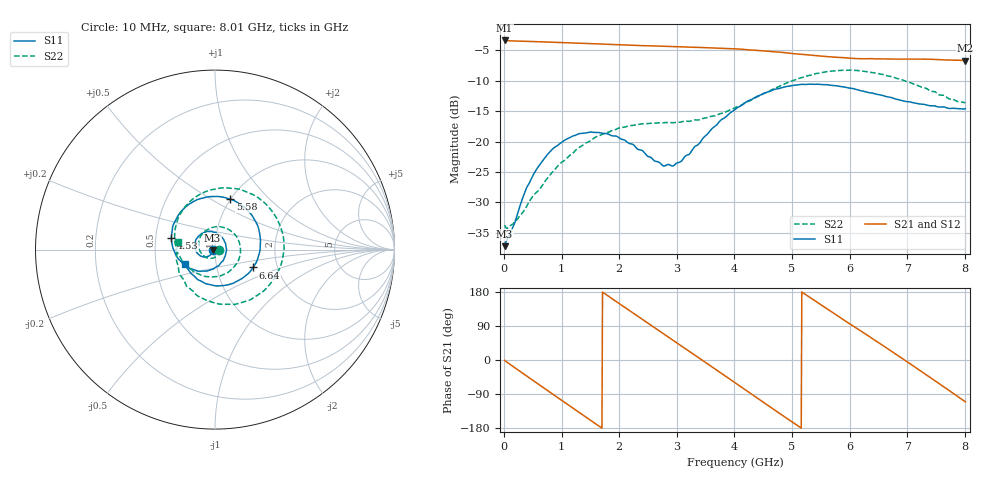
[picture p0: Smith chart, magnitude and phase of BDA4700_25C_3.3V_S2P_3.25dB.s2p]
!Agilent Technologies,E5071B,MY42404982,A.09.10
!Date: Mon Oct 20 18:04:20 2025
!Data & Calibration Information:
!Freq	S11:SOLT2(ON)	S21:SOLT2(ON)	S12:SOLT2(ON)	S22:SOLT2(ON)
# Hz S RI R 50
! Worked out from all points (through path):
!   801 points, 10 MHz to 8.01 GHz, reference 50 ohm
!   highest |S21| = -3.37 dB at 10 MHz (marker M1); lowest = -6.7 dB at 8.01 GHz (marker M2)
!   group delay of S21, straight-line fit = 287 ps
!   lowest |S11| = -37.2 dB at 10 MHz (marker M3), VSWR 1.03, Z = 48.6 - j0.153 ohm
!   |S11| at or under -10 dB: start of sweep to end of sweep
!   |S22| runs from -34.3 to -8.2 dB; largest |S21 - S12| = 0.0077
!   S11 on the Smith chart (normalised r, x): 10 MHz: 0.97, -0.00; 4.53 GHz: 0.60, +0.08; 5.58 GHz: 1.00, +0.61; 6.64 GHz: 1.50, -0.32; 8.01 GHz: 0.70, -0.12
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1e7  -0.0137 -0.00158  0.6786 -0.0146  0.6784 -0.0151  0.0205 -0.0018
3.3e8  -0.0228 -0.0266  0.5442 -0.3886  0.5438 -0.3889  0.019 -0.0182
7.1e8  -0.061 -0.041  0.1621 -0.6395  0.1619 -0.6396  -0.00785 -0.0462
1.02e9  -0.0981 -0.0206  -0.2065 -0.6184  -0.2065 -0.6187  -0.0548 -0.041
1.35e9  -0.1134 0.0279  -0.5151 -0.3859  -0.5155 -0.3861  -0.0908 0.0153
1.92e9  -0.0508 0.0989  -0.5789 0.2436  -0.5793 0.2436  -0.00898 0.1247
2.31e9  0.0168 0.0857  -0.2783 0.5514  -0.278 0.5515  0.0993 0.0953
2.68e9  0.059 0.0336  0.1221 0.5979  0.1216 0.5972  0.142 -0.0117
3.06e9  0.0541 -0.0413  0.4688 0.3775  0.4649 0.381  0.0877 -0.115
3.36e9  0.0137 -0.0927  0.5895 0.0824  0.5904 0.0825  0.00419 -0.1503
3.67e9  -0.0604 -0.1196  0.5353 -0.2425  0.5353 -0.2437  -0.0897 -0.1364
4.01e9  -0.1574 -0.0946  0.2896 -0.5009  0.2904 -0.5002  -0.1752 -0.073
4.53e9  -0.2435 0.0636  -0.2298 -0.5065  -0.2293 -0.5071  -0.2219 0.1168
4.94e9  -0.1827 0.2196  -0.4921 -0.2082  -0.492 -0.2112  -0.1226 0.2827
5.35e9  -0.0193 0.2955  -0.4847 0.1673  -0.4856 0.1645  0.0951 0.3409
5.58e9  0.0862 0.2805  -0.3718 0.3365  -0.3721 0.3361  0.2262 0.2984
6.09e9  0.242 0.1218  0.0264 0.4816  0.0277 0.4835  0.3838 0.0342
6.64e9  0.2117 -0.0994  0.4063 0.2522  0.4066 0.2515  0.2442 -0.2491
6.68e9  0.2027 -0.1133  0.4224 0.2229  0.4232 0.2219  0.2238 -0.2629
7.24e9  0.0247 -0.2018  0.415 -0.2355  0.4141 -0.2359  -0.0632 -0.2746
7.63e9  -0.0958 -0.1675  0.1584 -0.4427  0.1579 -0.4434  -0.1978 -0.1368
8.01e9  -0.1673 -0.0824  -0.1611 -0.4349  -0.1595 -0.4356  -0.2048 0.041
